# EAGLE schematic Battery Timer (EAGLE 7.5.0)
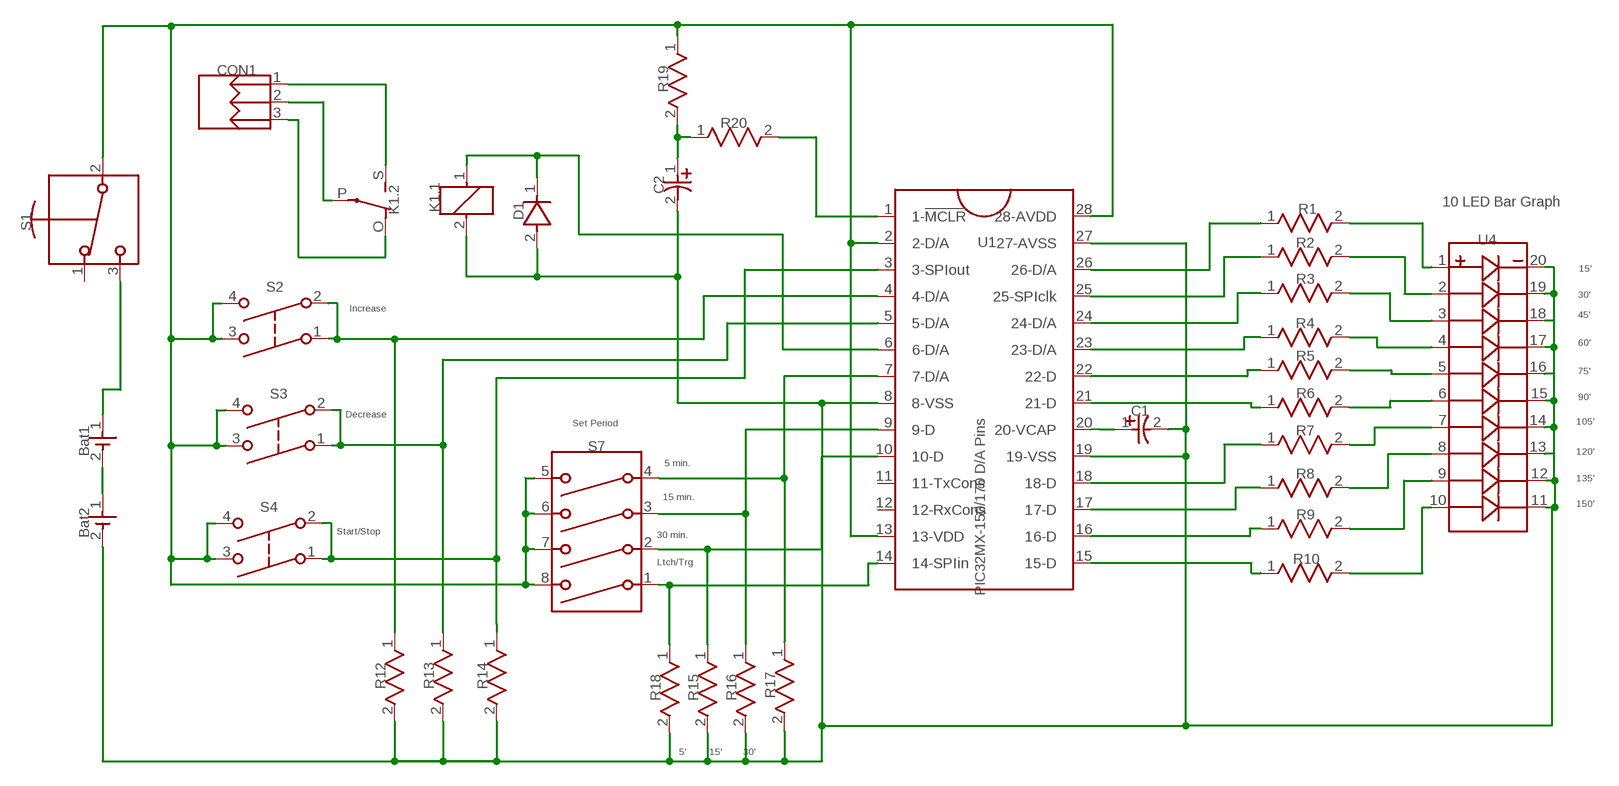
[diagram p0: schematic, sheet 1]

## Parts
Bat1  1025  [2466]
Bat2  1025  [2466]
C1  47UF  [CAP_1206]
C2  47uF  DEV_C2  [CAPR-2.5/6.5H12]
CON1  644456-3  [SHDRV3W125P500_3X1_1500X830H1240]
D1  DIODE  [DIO_1206]
K1  351  [ZF112]
R1  320  RES  [RES_1206]
R2  320  RES  [RES_1206]
R3  320  RES  [RES_1206]
R4  320  RES  [RES_1206]
R5  320  RES  [RES_1206]
R6  320  RES  [RES_1206]
R7  320  RES  [RES_1206]
R8  320  RES  [RES_1206]
R9  320  RES  [RES_1206]
R10  320  RES  [RES_1206]
R12  1K  RES  [RES_1206]
R13  1K  RES  [RES_1206]
R14  1K  RES  [RES_1206]
R15  1K  RES  [RES_1206]
R16  1K  RES  [RES_1206]
R17  1K  RES  [RES_1206]
R18  1K  RES  [RES_1206]
R19  50K  RES  [RES_1206]
R20  1K  RES  [RES_1206]
S1  JS102011SCQN  [CK_GS01MCBE]
S2  SWITCH_DPST_NO  [B3F-1]
S3  SWITCH_DPST_NO  [B3F-1]
S4  SWITCH_DPST_NO  [B3F-1]
S7  BD04  [BD04]
U1  PIC32MX-D/A_28PINS  [DIP-28]
U4  10LED_BAR  [10LED_BAR]

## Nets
Net_0: R1.1(A) U1.26(26-D/A)
Net_1: R2.1(A) U1.25(25-SPIclk)
Net_2: R3.1(A) U1.24(24-D/A)
Net_3: R4.1(A) U1.23(23-D/A)
Net_4: R5.1(A) U1.22(22-D)
Net_5: R6.1(A) U1.21(21-D)
Net_6: R10.1(A) U1.15(15-D)
Net_7: R9.1(A) U1.16(16-D)
Net_8: R8.1(A) U1.17(17-D)
Net_9: R7.1(A) U1.18(18-D)
Net_10: C1.1(PLUS) U1.20(20-VCAP)
Net_11: R18.1(A) S7.1 U1.14(14-SPIin)
Net_12: R19.1(A) S1.2(COMM) S2.3(C2) S2.4(C4) S3.3(C2) S3.4(C4) S4.3(C2) S4.4(C4) S7.5 S7.6 S7.7 S7.8 U1.2(2-D/A) U1.13(13-VDD) U1.28(28-AVDD)
Net_13: R10.2(B) U4.10
Net_14: R9.2(B) U4.9
Net_15: Bat2.2(NEG) C1.2(MINUS) C2.2(MINUS) D1.2(A) K1.2 R12.2(B) R13.2(B) R14.2(B) R15.2(B) R16.2(B) R17.2(B) R18.2(B) U1.8(8-VSS) U1.19(19-VSS) U1.27(27-AVSS) U4.11 U4.12 U4.13 U4.14 U4.15 U4.16 U4.17 U4.18 U4.19 U4.20
Net_16: R8.2(B) U4.8
Net_17: R7.2(B) U4.7
Net_18: R6.2(B) U4.6
Net_19: R4.2(B) U4.4
Net_20: R3.2(B) U4.3
Net_21: R2.2(B) U4.2
Net_22: R1.2(B) U4.1
Net_23: Bat1.1(POS) S1.3
Net_24: R12.1(A) S2.1(C1) S2.2(C3) U1.4(4-D/A)
Net_25: R13.1(A) S3.1(C1) S3.2(C3) U1.5(5-D/A)
Net_26: R14.1(A) S4.1(C1) S4.2(C3) U1.3(3-SPIout)
Net_27: CON1.1 K1.S(PART_2:S)
Net_28: Bat1.2(NEG) Bat2.1(POS)
Net_29: D1.1(K) K1.1 U1.6(6-D/A)
Net_30: CON1.2 K1.P(PART_2:P)
Net_31: CON1.3 K1.O(PART_2:O)
Net_32: R15.1(A) S7.2 U1.10(10-D)
Net_33: R5.2(B) U4.5
Net_34: R20.2(B) U1.1(1-!MCLR!)
Net_35: R17.1(A) S7.4 U1.7(7-D/A)
Net_36: R16.1(A) S7.3 U1.9(9-D)
Net_37: C2.1(PLUS) R19.2(B) R20.1(A)
Unconnected: S1.1 U1.11(11-TxCons) U1.12(12-RxCons)

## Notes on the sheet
- CON1
- R19
- R20
- C2 | 10 LED Bar Graph
- S1 | K1.2 | K1.1 | R1
- D1
- U1 | R2 | U4
- 15'
- R3
- S2 | 30'
- Increase
- 45'
- R4
- 60'
- R5
- 75'
- 90'
- S3 | R6
- Decrease
- C1 | 105'
- Set Period
- R7
- 120'
- S7
- Bat1
- 5 min.
- 135'
- R8
- 15 min.
- 150'
- S4
- R9
- Start/Stop
- 30 min.
- Bat2
- Ltch/Trg
- R10
- PIC32MX-150/170 D/A Pins
- R12 | R13 | R14
- R18 | R15 | R16 | R17
- 5' | 15' | 30'

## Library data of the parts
Bat1 Bat2 = common:1025; DATASHEET: http://datasheets.diptrace.com/con_batteries/1025.pdf; MANUFACTURER: Keystone
C1 = common:47UF
C2 = common:DEV_C2; DATASHEET: http://datasheets.diptrace.com/cap/eeefk.pdf; MANUFACTURER: Panasonic
CON1 = common:644456-3; DATASHEET: http://datasheets.diptrace.com/con_headers/ENG_CD_644456_D2.pdf; MANUFACTURER: TE Connectivity
D1 = common:DIODE
K1 = common:351
R1-R10 = common:RES
R12-R20 = common:RES; VALUE: 320
S1 = common:JS102011SCQN; DATASHEET: http://datasheets.diptrace.com/switches/JS_series.pdf; MANUFACTURER: C&K
S2-S4 = common:SWITCH_DPST_NO; DESCRIPTION: Switch; UNTITLED: Normally Open
S7 = common:BD04; DATASHEET: http://datasheets.diptrace.com/switches/BD_series.pdf; MANUFACTURER: C&K
U1 = common:PIC32MX-D/A_28PINS; MANUFACTURER: MICROMITE
U4 = common:10LED_BAR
